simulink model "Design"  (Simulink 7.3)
settings: Solver=ode45  StartTime=0.0  StopTime=10.0  RelTol=1e-3
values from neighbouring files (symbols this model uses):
  Kp = om^2    (= 1.44)    [run.m]
  Kr = 2*zt*om    (= 0.336)    [run.m]
  Q = diag([0.09, 0.12, 0.001, 0.1, 0.001, 0.1, 0.24, 0.13, 0.07])    [run.m]
undefined symbols (not defined in the file or in its folder): Ad, Bd, Cd, Dd

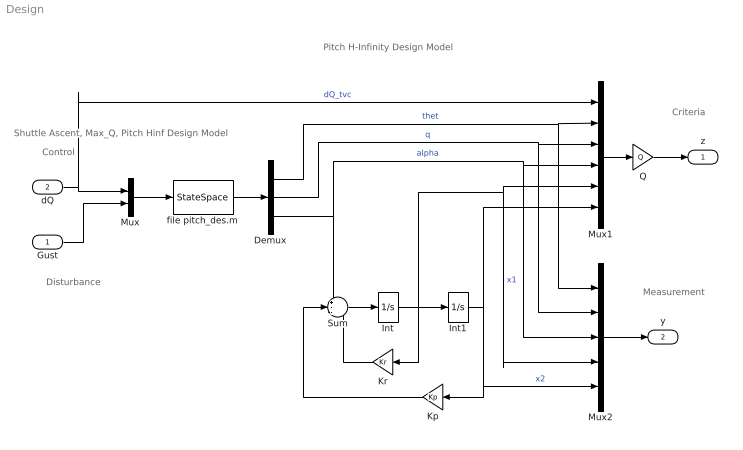
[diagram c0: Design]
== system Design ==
  note: Shuttle Ascent, Max_Q, Pitch Hinf Design Model
  note: Pitch H-Infinity Design Model
  note: Criteria
  note: Measurement
  note: Disturbance
  note: Control
  Gust : Inport  OutDataType=sfix(16)  OutScaling=2^0
  dQ : Inport  Port=2  OutDataType=sfix(16)  OutScaling=2^0
  Demux : Demux  Outputs=3
  Int : Integrator
  Int1 : Integrator
  Kp : Gain  Gain=Kp  ParameterDataType=sfix(16)  ParameterScaling=2^0  OutDataType=sfix(16)  OutScaling=2^0
  Kr : Gain  Gain=Kr  ParameterDataType=sfix(16)  ParameterScaling=2^0  OutDataType=sfix(16)  OutScaling=2^0
  Mux : Mux  Inputs=2
  Mux1 : Mux  Inputs=6
  Mux2 : Mux  Inputs=5
  Q : Gain  Gain=Q  Multiplication=Matrix(K*u)  ParameterDataType=sfix(16)  ParameterScaling=2^0  OutDataType=sfix(16)  OutScaling=2^0
  Sum : Sum  Inputs=+--  OutDataType=sfix(16)  OutScaling=2^0
  file pitch_des.m : StateSpace  A=Ad  B=Bd  C=Cd  D=Dd
  z : Outport  OutDataType=sfix(16)  OutScaling=2^0
  y : Outport  Port=2  OutDataType=sfix(16)  OutScaling=2^0
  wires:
  file pitch_des.m/1 -> Demux/1
  Mux/1 -> file pitch_des.m/1
  Demux/1 -> Mux1/2, Mux2/1  "thet"
  dQ/1 -> Mux/1, Mux1/1  "dQ_tvc"
  Demux/2 -> Mux1/3, Mux2/2  "q"
  Int/1 -> Int1/1, Kr/1, Mux1/5, Mux2/4  "x1"
  Sum/1 -> Int/1
  Int1/1 -> Kp/1, Mux2/5, Mux1/6  "x2"
  Kr/1 -> Sum/3
  Kp/1 -> Sum/2
  Demux/3 -> Sum/1, Mux1/4, Mux2/3  "alpha"
  Gust/1 -> Mux/2
  Mux1/1 -> Q/1
  Mux2/1 -> y/1
  Q/1 -> z/1
